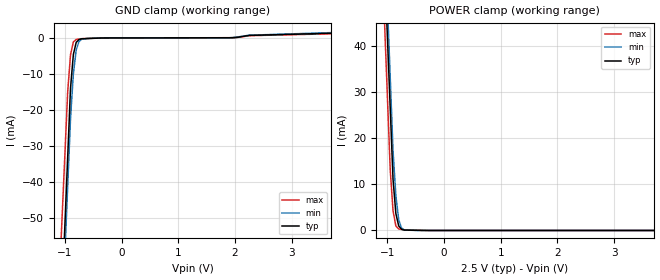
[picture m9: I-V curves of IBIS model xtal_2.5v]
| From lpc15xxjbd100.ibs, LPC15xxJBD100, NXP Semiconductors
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[Model] xtal_2.5v
Model_type Input
Vinl = 750.000mV
Vinh = 1.75000V
C_comp 1.24000pF 1.24000pF 1.24000pF
| variable typ   min   max
[Voltage Range] 2.50000V 2.25000V 2.75000V
[POWER Clamp Reference] 2.50000V 2.25000V 2.75000V
[GND Clamp Reference] 0.00000V 0.00000V 0.00000V
[Temperature Range]   25   85   -40
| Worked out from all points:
|   GND clamp passes 1 mA (typ) near -0.78 V on its own axis
|   POWER clamp passes 1 mA (typ) near -0.80 V on its own axis
[GND Clamp]
-2.5V     -627.1mA   -626.3mA   -562.6mA
-950mV    -33.09mA   -41.24mA   -14.93mA
-900mV    -13.92mA   -22.37mA   -4.663mA
-850mV    -4.63mA    -9.99mA    -1.142mA
-800mV    -1.259mA   -3.372mA   -456.2uA
-750mV    -460.7uA   -994.5uA   -340.5uA
-700mV    -271.1uA   -396.2uA   -224.8uA
-600mV    -206uA     -156.1uA   -165.8uA
1.9V      24.31uA    19.27uA    29.46uA
2.25V     668.3uA    729.5uA    595.9uA
5V        1.817mA    2.093mA    1.594mA
[POWER Clamp]
-2.5V     507mA      528.7mA    505.9mA
-1.05V    57.58mA    65.22mA    45.02mA
-950mV    26.59mA    33.25mA    13.23mA
-900mV    11.09mA    17.27mA    4.268mA
-850mV    3.645mA    7.526mA    964.6uA
-800mV    995.8uA    2.355mA    319.3uA
-750mV    248.2uA    526uA      231.3uA
-700mV    90.11uA    99.83uA    143.4uA
-500mV    38.62uA    11.09uA    83.02uA
5V        0A         0A         0A
